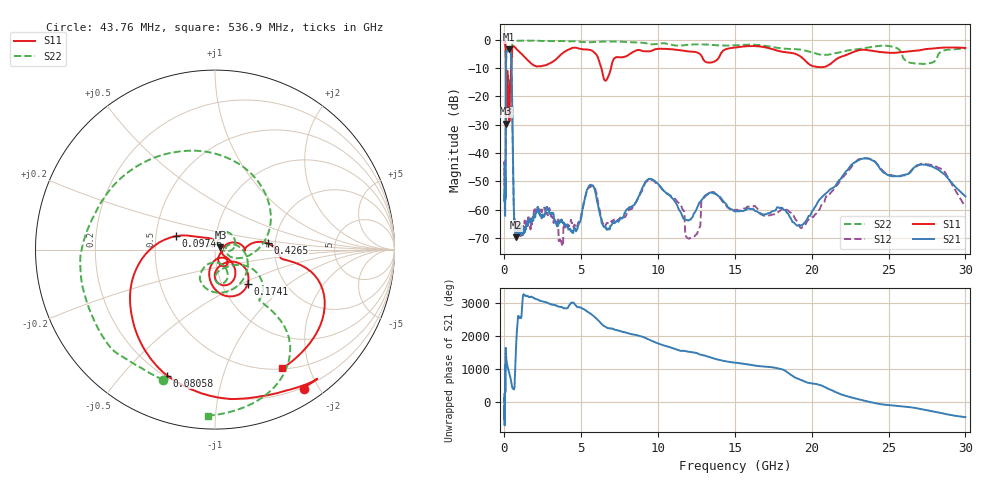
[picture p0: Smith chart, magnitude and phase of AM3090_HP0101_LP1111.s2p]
! Date/Time: Thu, Feb 28, 2019 1:59 PM
! Network Analyzer: Agilent Technologies E8364B Rev: A.07.50.67
! Sweep from 0.010 to 30.000 GHz, 1601 Points, Sweep Type: LOG
! Power Supply: 5.023 V, 0.002 A
# Hz S DB R 50
!freq MagS11 AngS11 MagS21 AngS21 MagS12 AngS12 MagS22 AngS22
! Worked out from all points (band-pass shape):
!   1601 points, 10 MHz to 30 GHz, reference 50 ohm
!   highest |S21| = -3.33 dB at 267.8 MHz (marker M1); lowest = -69.8 dB at 754.5 MHz (marker M2)
!   |S21| within 3 dB of the highest: 110.3 MHz to 441.7 MHz (331.4 MHz wide, 120 % of centre)
!   lowest |S11| = -29.6 dB at 105.1 MHz (marker M3), VSWR 1.07, Z = 53.1 + j1.34 ohm
!   |S11| at or under -10 dB: 95.94 MHz to 430 MHz (334 MHz wide, 127 % of centre); 6.308 GHz to 6.931 GHz (622.6 MHz wide, 9.4 % of centre)
!   |S22| runs from -30.8 to -0.2 dB; largest |S21 - S12| = 0.0081
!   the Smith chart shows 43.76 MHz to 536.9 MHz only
!   S11 on the Smith chart (normalised r, x): 43.76 MHz: 0.18, -1.81; 80.58 MHz: 0.21, -0.67; 97.46 MHz: 0.64, +0.10; 174.1 MHz: 1.32, -0.54; 426.5 MHz: 1.83, +0.14; 536.9 MHz: 0.51, -1.60
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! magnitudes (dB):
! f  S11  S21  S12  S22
! 10 MHz  -0.2  -43.7  -43.3  -0.7
! 38.04 MHz  -0.5  -59.9  -59.4  -1.7
! 43.76 MHz  -0.7  -60.6  -57.9  -2.1
! 80.58 MHz  -2.5  -49.2  -48.5  -4.5
! 97.46 MHz  -12.7  -15.3  -15.2  -13.5
! 105.1 MHz  -29.6  -8.0  -8.0  -30.6
! 144.7 MHz  -20.7  -3.8  -3.8  -24.3
! 174.1 MHz  -11.6  -3.6  -3.5  -14.3
! 267.8 MHz  -21.0  -3.3  -3.3  -18.1
! 426.5 MHz  -10.6  -5.4  -5.4  -10.6
! 536.9 MHz  -2.4  -38.1  -38.2  -0.7
! 550.5 MHz  -2.3  -42.7  -42.8  -0.5
! 754.5 MHz  -3.0  -69.8  -65.4  -0.3
! 2.084 GHz  -9.4  -60.8  -60.5  -0.3
! 3.668 GHz  -5.2  -64.4  -71.2  -0.4
! 7.926 GHz  -5.8  -60.2  -62.0  -0.7
! 9.538 GHz  -4.0  -49.1  -49.5  -1.5
! 12.25 GHz  -4.2  -62.6  -69.9  -1.6
! 13.4 GHz  -8.0  -54.0  -53.8  -1.7
! 19.51 GHz  -7.0  -64.7  -65.9  -3.7
! 23.48 GHz  -3.5  -41.8  -41.9  -2.9
! 30 GHz  -2.8  -55.3  -58.9  -3.1
